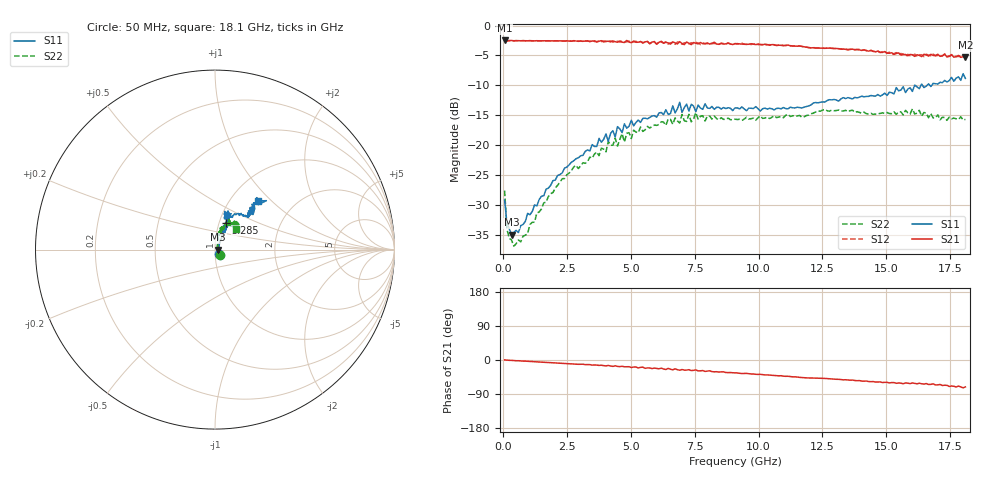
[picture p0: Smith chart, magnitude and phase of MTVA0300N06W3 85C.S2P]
! Network Analyzer HP8720D.06.14 Serial No. US36140669
!  7 Jul 2005  10:24:06
! Frequency  S11  S21  S12  S22
# HZ  S  DB R 50
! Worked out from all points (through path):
!   201 points, 50 MHz to 18.1 GHz, reference 50 ohm
!   highest |S21| = -2.50 dB at 50 MHz (marker M1); lowest = -5.3 dB at 18.1 GHz (marker M2)
!   group delay of S21, straight-line fit = 11 ps
!   lowest |S11| = -35.0 dB at 320.8 MHz (marker M3), VSWR 1.04, Z = 51.8 - j0.0766 ohm
!   |S11| at or under -10 dB: start of sweep to 16.11 GHz; 16.13 GHz to 16.36 GHz (234.6 MHz wide, 1.44 % of centre); 16.42 GHz to 16.6 GHz (184.2 MHz wide, 1.12 % of centre)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
!   |S22| runs from -36.9 to -13.9 dB; largest |S21 - S12| = 0.038
!   S11 on the Smith chart (normalised r, x): 50 MHz: 1.04, -0.06; 5.285 GHz: 1.07, +0.33; 18.1 GHz: 1.33, +0.83
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5e7  -29.22 -50.4  -2.50 0.3  -2.52 0.3  -27.62 -47.1
1.4025e8  -33.02 -29.9  -2.58 -0.3  -2.56 -0.4  -34.08 -33.8
3.2075e8  -35.01 -2.4  -2.50 -0.9  -2.53 -0.9  -35.91 -7.2
6.8175e8  -33.50 25.5  -2.55 -2.5  -2.54 -2.6  -36.22 29.5
2.30625e9  -24.68 57.1  -2.58 -8.4  -2.57 -8.6  -25.65 72.0
3.1185e9  -21.73 62.8  -2.63 -11.1  -2.65 -11.5  -22.98 75.6
4.021e9  -18.15 65.4  -2.64 -15.5  -2.67 -14.5  -21.14 72.6
4.11125e9  -19.37 65.6  -2.63 -14.4  -2.70 -15.7  -19.39 72.7
4.47225e9  -16.93 61.6  -2.80 -16.8  -2.61 -15.9  -20.20 77.3
4.65275e9  -17.93 62.0  -2.79 -16.5  -2.64 -17.9  -18.09 76.5
4.743e9  -16.46 65.3  -2.84 -18.0  -2.75 -17.0  -19.50 72.8
5.2845e9  -15.83 68.5  -2.80 -21.0  -2.85 -20.3  -17.95 66.6
6.09675e9  -14.64 67.1  -2.80 -23.2  -2.71 -23.0  -16.57 66.8
6.7285e9  -14.62 74.3  -2.89 -23.3  -3.15 -24.3  -15.47 60.9
6.909e9  -12.84 71.4  -2.70 -26.9  -2.81 -25.2  -16.33 61.0
6.99925e9  -14.53 71.1  -3.00 -25.1  -3.14 -27.3  -14.89 61.9
7.17975e9  -13.15 75.7  -2.75 -26.6  -3.03 -25.4  -16.06 57.6
7.54075e9  -14.41 68.5  -2.97 -26.2  -2.82 -29.0  -14.59 65.2
9.075e9  -13.78 72.3  -3.04 -33.8  -3.02 -34.0  -15.68 55.7
1.21435e10  -12.98 61.3  -3.71 -47.3  -3.67 -47.4  -14.66 56.1
1.512175e10  -11.16 44.5  -4.64 -60.6  -4.45 -59.9  -14.74 52.0
1.81e10  -8.85 48.5  -5.33 -71.0  -5.56 -72.2  -15.72 44.5
